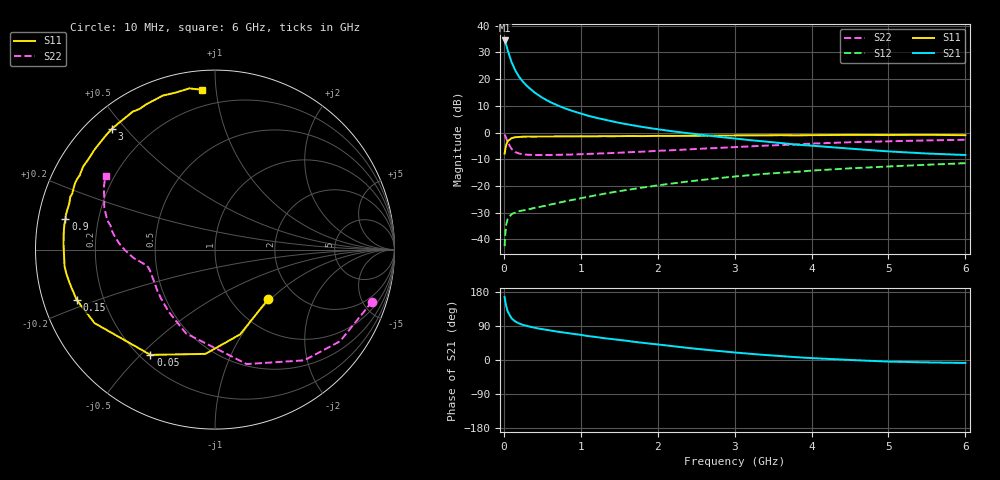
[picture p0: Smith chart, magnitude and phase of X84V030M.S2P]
! SIEMENS Small Signal Semiconductors
! BFP136W
! Si NPN RF Bipolar Junction Transistor in SOT343
! VCE = 4 V  IC = 30 mA
! Common Emitter S-Parameters:  September  1994
# GHz  S  MA  R  50
!  f  S11  S21  S12  S22
! GHz  MAG  ANG  MAG  ANG  MAG  ANG  MAG  ANG
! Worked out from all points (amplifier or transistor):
!   40 points, 10 MHz to 6 GHz, reference 50 ohm
!   highest |S21| = 34.5 dB at 10 MHz (marker M1)
!   |S21| within 3 dB of that: start of sweep to 43.71 MHz
!   unconditionally stable (mu >= 1): 808.9 MHz to 2.801 GHz
!   at 200 MHz: K = 0.42, MSG = 25.1 dB, |S12| = -29.4 dB
!   at 1.5 GHz: K = 1.12, MAG = 10.6 dB, |S12| = -21.9 dB
!   at 6 GHz: K = 0.96, MSG = 1.5 dB, |S12| = -11.4 dB
!   S11 on the Smith chart (normalised r, x): 10 MHz: 1.47, -0.96; 50 MHz: 0.24, -0.54; 150 MHz: 0.10, -0.17; 900 MHz: 0.08, +0.10; 3 GHz: 0.07, +0.46; 6 GHz: 0.10, +0.92
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0.01  0.4048 -42.6  52.97 166.3  0.0075 75.6  0.9218 -18.3
0.02  0.4926 -73.5  48.54 153.6  0.0134 65.7  0.8641 -36.2
0.03  0.5834 -95.2  44.24 143.3  0.0187 56.0  0.7927 -51.1
0.05  0.6879 -121.5  34.75 128.2  0.0245 43.2  0.6618 -74.5
0.1  0.7862 -148.6  20.87 110.0  0.0299 31.7  0.4942 -109.0
0.15  0.8198 -160.0  14.51 101.5  0.0319 29.5  0.4308 -127.1
0.2  0.8294 -166.2  10.99 96.3  0.0339 29.0  0.4054 -138.0
0.25  0.8387 -170.6  8.894 92.6  0.0351 29.3  0.3935 -145.1
0.3  0.8433 -173.6  7.457 89.9  0.036 30.5  0.3854 -150.0
0.4  0.8419 -178.6  5.623 85.1  0.0391 33.7  0.3808 -156.4
0.5  0.8444 178.0  4.49 81.3  0.0416 36.7  0.3798 -160.3
0.6  0.8462 175.4  3.744 78.2  0.0449 39.4  0.3812 -162.7
0.7  0.849 172.6  3.224 74.7  0.0482 42.2  0.3837 -164.3
0.9  0.8501 168.5  2.521 69.0  0.0553 46.0  0.3897 -166.8
1.1  0.8514 163.8  2.059 63.0  0.0631 49.1  0.3994 -168.1
1.5  0.8582 156.9  1.524 53.0  0.0802 52.4  0.4204 -170.6
2.2  0.8669 144.3  1.054 36.4  0.1122 52.3  0.4689 -175.8
3  0.8847 130.4  0.777 19.9  0.1507 47.9  0.5353 176.3
3.2  0.8861 127.0  0.723 16.4  0.1598 46.4  0.5519 173.9
4.5  0.9059 108.6  0.501 0.1  0.2143 35.2  0.6601 159.1
5.5  0.9098 99.1  0.406 -6.3  0.2503 27.2  0.7149 149.9
6  0.8937 94.7  0.381 -7.8  0.2678 22.8  0.7345 146.0
